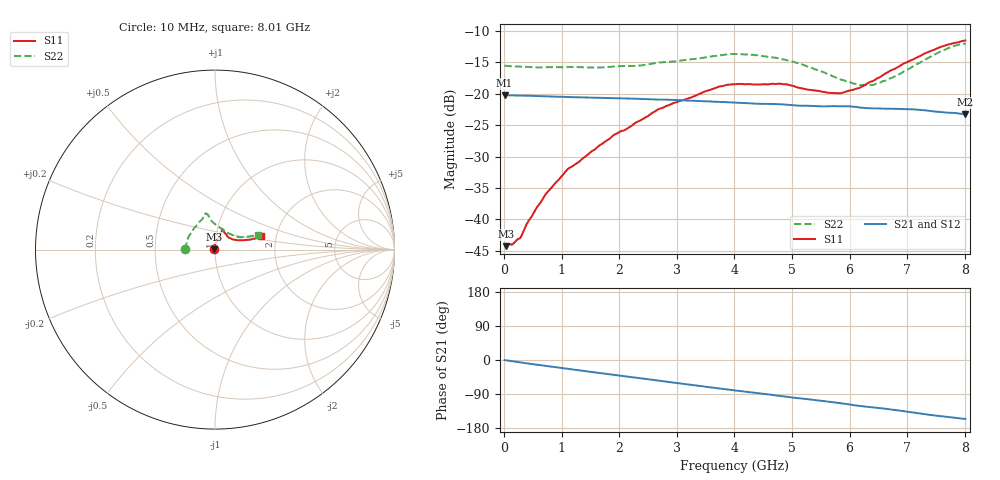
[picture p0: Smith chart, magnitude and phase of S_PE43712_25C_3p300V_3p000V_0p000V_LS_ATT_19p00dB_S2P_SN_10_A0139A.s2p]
! DEVICE ID: PE43712
! File Path: z:\PE43713\PE43713_CHAR_NOM_04292014\AMB\3p300\LS_ATT_19p00dB\PE43713_AMB_3p300V_3p000V_0p000V_LS_ATT_19p00dB_S2P_SN_10_A0139A.s2p
! Serial: 10
! Lot: A0139A
! Temp: 25C
! VDD: 3.300
! VSS: 0.000
! Control_Hi: 3.000
! Control_Lo: 0.000
! Attenuation Step: 19.00dB
! Port 1: RF1
! Port 2: RF2
! ThroughPath:1-2
! IDD: 0.0001467957
! ISS: -2.99e-008
#  Hz  S  RI  R  50
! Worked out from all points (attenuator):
!   801 points, 10 MHz to 8.01 GHz, reference 50 ohm
!   highest |S21| = -20.22 dB at 10 MHz (marker M1); lowest = -23.3 dB at 8 GHz (marker M2)
!   lowest |S11| = -44.3 dB at 30 MHz (marker M3), VSWR 1.01, Z = 49.4 + j0.137 ohm
!   |S11| at or under -10 dB: start of sweep to end of sweep
!   |S22| runs from -18.7 to -12.0 dB; largest |S21 - S12| = 0.00036
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1e7  -0.00631 0.000566  0.0974 -0.000497  0.0975 -0.000497  -0.1675 0.0012
3e7  -0.00593 0.00138  0.0974 -0.00123  0.0974 -0.00125  -0.1669 0.00293
1.5e8  -0.0051 0.00372  0.097 -0.00578  0.097 -0.0058  -0.1654 0.011
2.7e8  -0.0044 0.00548  0.0963 -0.0102  0.0963 -0.0102  -0.1638 0.0176
4.2e8  -0.00405 0.00869  0.0953 -0.0156  0.0952 -0.0156  -0.1618 0.026
7.4e8  -0.00372 0.0158  0.0918 -0.0263  0.0918 -0.0263  -0.1567 0.0458
1.1e9  -0.00234 0.0249  0.0866 -0.0373  0.0867 -0.0373  -0.1488 0.0667
1.35e9  7.6e-05 0.0301  0.0826 -0.0443  0.0826 -0.0443  -0.1422 0.0794
1.91e9  0.00879 0.0462  0.0715 -0.0584  0.0715 -0.0584  -0.1218 0.1119
2.34e9  0.0181 0.0578  0.0613 -0.0676  0.0613 -0.0676  -0.1026 0.1327
2.68e9  0.0269 0.0705  0.0525 -0.073  0.0525 -0.073  -0.0863 0.1556
3.71e9  0.039 0.1062  0.023 -0.0831  0.023 -0.0831  -0.0558 0.1937
4.01e9  0.0402 0.1125  0.0144 -0.0839  0.0144 -0.0839  -0.0534 0.201
4.79e9  0.0438 0.1123  -0.00694 -0.0822  -0.00693 -0.0823  -0.0365 0.1875
5.35e9  0.0563 0.0908  -0.0206 -0.0773  -0.0206 -0.0773  -0.0191 0.1594
5.82e9  0.0738 0.0691  -0.0319 -0.0728  -0.0318 -0.0729  0.0143 0.1306
6.18e9  0.0961 0.0574  -0.0403 -0.0664  -0.0402 -0.0665  0.0497 0.1063
6.4e9  0.1137 0.0546  -0.0436 -0.0629  -0.0435 -0.0629  0.0738 0.0914
6.68e9  0.1413 0.0519  -0.0487 -0.0584  -0.0486 -0.0584  0.1063 0.0767
7.54e9  0.2243 0.0618  -0.0605 -0.0385  -0.0604 -0.0384  0.1996 0.0747
8e9  0.2549 0.0754  -0.0624 -0.0286  -0.0623 -0.0287  0.2368 0.0833
8.01e9  0.2554 0.0761  -0.0624 -0.0285  -0.0623 -0.0286  0.2374 0.0833
